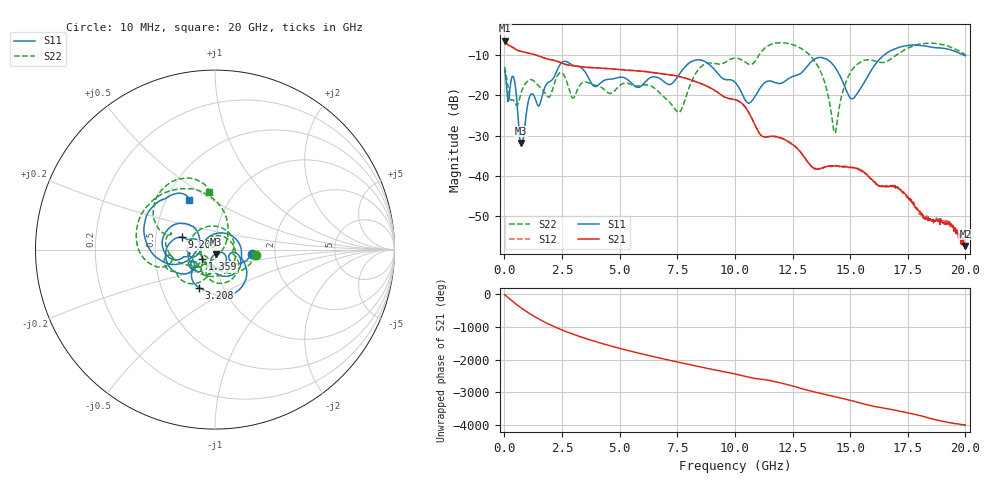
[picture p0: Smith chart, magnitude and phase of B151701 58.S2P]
!  2-Port S-parameters saved by WinCal
! VAR MeasName=S-Parameters (CALIBRATED_DATA) read from VNA (N5244A)
! VAR MeasDate=2015-12-24 19:16:51
! VAR NAME=B151701 58
! VAR FILENAME=B151701 58.S2P
! VAR DATE=2015-12-24 19:16:51
! VAR PHYS_PORTS=1,3
# Hz S DB R 50
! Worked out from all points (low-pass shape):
!   801 points, 10 MHz to 20 GHz, reference 50 ohm
!   highest |S21| = -6.31 dB at 10 MHz (marker M1); lowest = -57.6 dB at 20 GHz (marker M2)
!   |S21| within 3 dB of the highest: start of sweep to 961.1 MHz
!   lowest |S11| = -31.8 dB at 709.6 MHz (marker M3), VSWR 1.05, Z = 50.6 - j2.49 ohm
!   |S11| at or under -10 dB: start of sweep to 16.45 GHz; 19.96703 GHz to end of sweep
!   |S22| runs from -29.4 to -6.8 dB; largest |S21 - S12| = 0.0015
!   S11 on the Smith chart (normalised r, x): 10 MHz: 1.51, -0.07; 1.359 GHz: 0.86, -0.09; 3.208 GHz: 0.77, -0.34; 9.205 GHz: 0.68, +0.10; 20 GHz: 0.65, +0.40
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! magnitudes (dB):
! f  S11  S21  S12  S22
! 10 MHz  -13.7  -6.3  -6.3  -12.9
! 409.8 MHz  -15.7  -8.2  -8.2  -21.3
! 709.6 MHz  -31.8  -9.0  -9.0  -19.6
! 1.109 GHz  -20.1  -9.5  -9.5  -16.1
! 1.359 GHz  -21.2  -9.9  -9.9  -16.8
! 1.934 GHz  -16.6  -11.0  -11.0  -20.4
! 2.509 GHz  -11.7  -12.0  -12.0  -14.4
! 3.208 GHz  -12.8  -12.7  -12.7  -18.1
! 3.358 GHz  -13.2  -12.9  -12.9  -16.9
! 3.933 GHz  -17.8  -13.1  -13.1  -17.4
! 6.682 GHz  -15.6  -14.5  -14.5  -19.0
! 7.581 GHz  -14.8  -15.3  -15.2  -24.2
! 8.406 GHz  -11.1  -16.8  -16.8  -13.6
! 9.205 GHz  -14.1  -19.0  -19.0  -12.1
! 10.01 GHz  -16.7  -21.1  -21.1  -10.7
! 10.63 GHz  -21.9  -24.5  -24.5  -12.3
! 11.88 GHz  -17.0  -30.4  -30.3  -6.9
! 13.35 GHz  -11.4  -37.8  -37.8  -10.6
! 14.33 GHz  -12.9  -37.6  -37.6  -29.4
! 15.13 GHz  -20.7  -38.0  -38.1  -13.3
! 16.68 GHz  -9.1  -42.8  -42.6  -11.2
! 20 GHz  -10.1  -57.6  -57.6  -9.8
